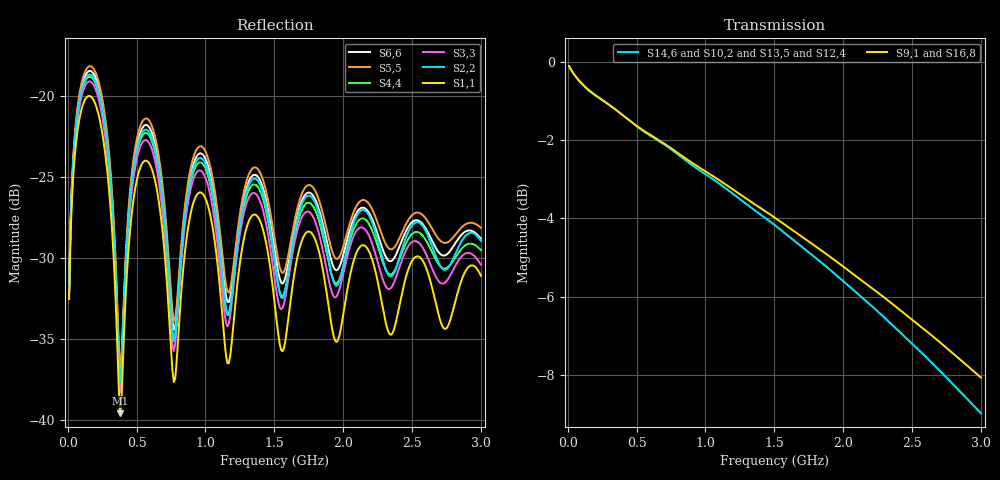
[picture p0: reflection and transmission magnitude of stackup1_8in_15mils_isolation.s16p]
! Touchstone file from project
# GHZ S RI R 50.000000
! Modal data exported
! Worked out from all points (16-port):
!   300 points, 10 MHz to 3 GHz, reference 50 ohm
!   strongest paths, dB at 10 MHz, 760 MHz, 1.51 GHz, 2.26 GHz, 3 GHz:
!     S9,1: -0.1, -2.2, -4.0, -5.9, -8.1
!     S16,8: -0.1, -2.3, -4.0, -5.9, -8.1
!     S14,6: -0.1, -2.3, -4.2, -6.4, -9.0
!     S10,2: -0.1, -2.3, -4.2, -6.4, -9.1
!     S13,5: -0.1, -2.3, -4.2, -6.4, -9.0
!     S12,4: -0.1, -2.3, -4.2, -6.4, -9.0
!   lowest |S11| = -39.6 dB at 380 MHz (marker M1), VSWR 1.02, Z = 50.9 - j0.506 ohm
!   |S11| at or under -10 dB: start of sweep to end of sweep
